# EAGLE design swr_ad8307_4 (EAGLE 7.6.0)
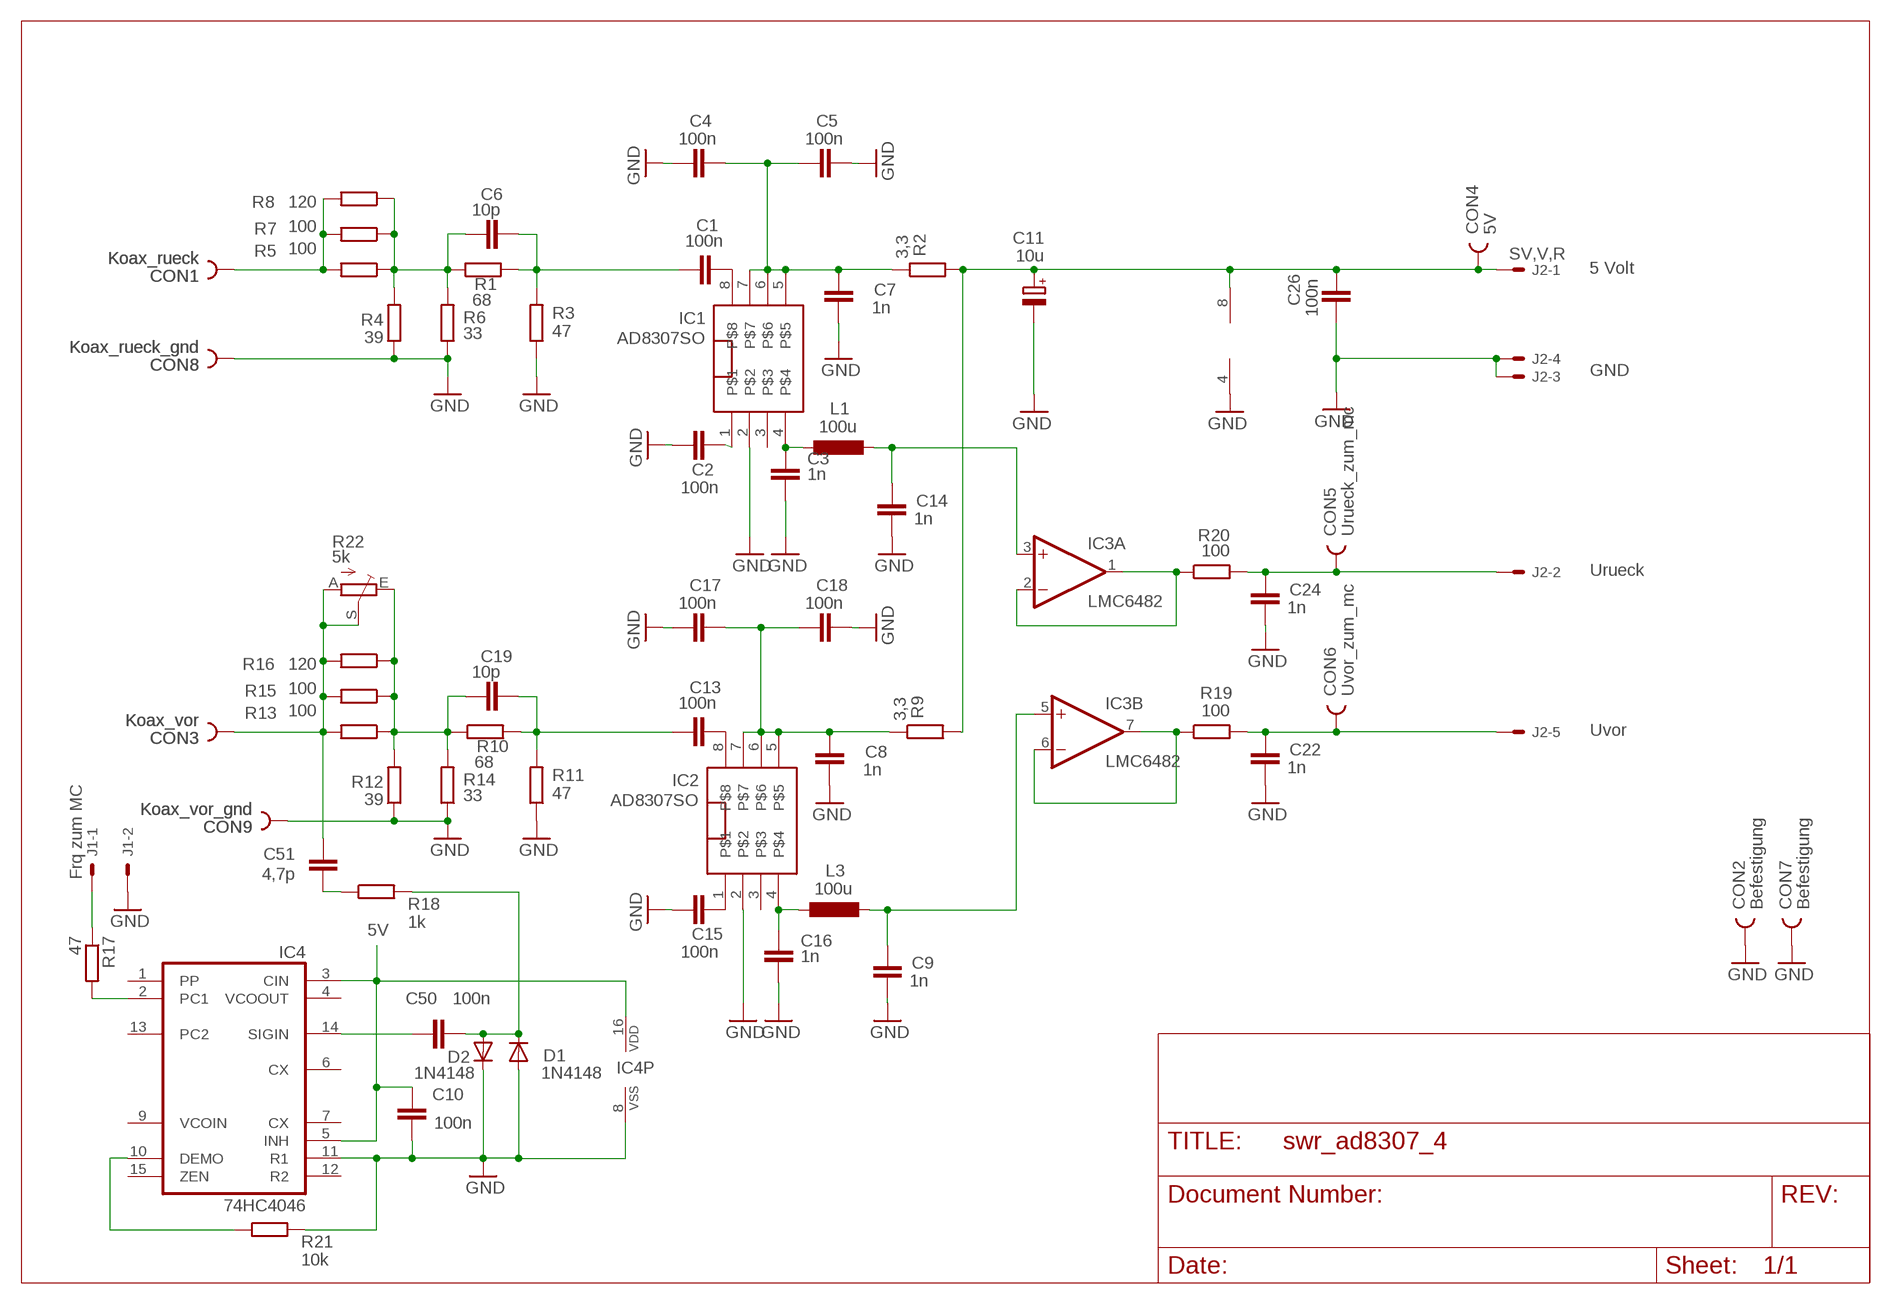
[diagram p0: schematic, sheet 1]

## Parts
C1  100n  C-EUC0805  [C0805]
C2  100n  C-EUC0805  [C0805]
C3  1n  C-EUC0805  [C0805]
C4  100n  C-EUC0805  [C0805]
C5  100n  C-EUC0805  [C0805]
C6  10p  C-EUC0805  [C0805]
C7  1n  C-EUC0805  [C0805]
C8  1n  C-EUC0805  [C0805]
C9  1n  C-EUC0805  [C0805]
C10  100n  C-EUC0805  [C0805]
C11  10u  CPOL-EUSMCB  [SMC_B]
C13  100n  C-EUC0805  [C0805]
C14  1n  C-EUC0805  [C0805]
C15  100n  C-EUC0805  [C0805]
C16  1n  C-EUC0805  [C0805]
C17  100n  C-EUC0805  [C0805]
C18  100n  C-EUC0805  [C0805]
C19  10p  C-EUC0805  [C0805]
C22  1n  C-EUC0805  [C0805]
C24  1n  C-EUC0805  [C0805]
C26  100n  C-EUC0805  [C0805]
C50  100n  C-EUC0805  [C0805]
C51  4,7p  C-EUC0805  [C0805]
CON1  Koax_rueck  PIN1_75OV  [PIN_1,75OV]
CON2  Befestigung  PIN2_53MM  [HOLE3]
CON3  Koax_vor  PIN1_75OV  [PIN_1,75OV]
CON4  5V  PIN1_75  [PIN1_75]
CON5  Urueck_zum_mc  PIN1_75  [PIN1_75]
CON6  Uvor_zum_mc  PIN1_75  [PIN1_75]
CON7  Befestigung  PIN2_53MM  [HOLE3]
CON8  Koax_rueck_gnd  PIN1_75OV  [PIN_1,75OV]
CON9  Koax_vor_gnd  PIN1_75OV  [PIN_1,75OV]
D1  1N4148  DIODE-SOD80C  [SOD80C]
D2  1N4148  DIODE-SOD80C  [SOD80C]
IC1  AD8307SO  [SO8]
IC2  AD8307SO  [SO8]
IC3  LMC6482  TL082D  [SO08]
IC4  74HC4046  4046D  [SO16]
J1  Frq zum MC  22-05-7028-02  [7395-02]
J2  SV,V,R  22-05-7058-05  [7395-05]
L1  100u  L-EUL3230M  [L3230M]
L3  100u  L-EUL3230M  [L3230M]
R1  68  R-EU_M0805  [M0805]
R2  3,3  R-EU_M0805  [M0805]
R3  47  R-EU_M0805  [M0805]
R4  39  R-EU_M0805  [M0805]
R5  100  R-EU_M1206  [M1206]
R6  33  R-EU_M0805  [M0805]
R7  100  R-EU_M1206  [M1206]
R8  120  R-EU_M1206  [M1206]
R9  3,3  R-EU_M0805  [M0805]
R10  68  R-EU_M0805  [M0805]
R11  47  R-EU_M0805  [M0805]
R12  39  R-EU_M0805  [M0805]
R13  100  R-EU_M1206  [M1206]
R14  33  R-EU_M0805  [M0805]
R15  100  R-EU_M1206  [M1206]
R16  120  R-EU_M1206  [M1206]
R17  47  R-EU_M0805  [M0805]
R18  1k  R-EU_M0805  [M0805]
R19  100  R-EU_M0805  [M0805]
R20  100  R-EU_M0805  [M0805]
R21  10k  R-EU_M0805  [M0805]
R22  5k  TRIM_EU-CA6H  [CA6H]

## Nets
5V: C10.2 C11.+ C26.1 CON4.1 IC3.8(P:V+) IC4.3(CIN) IC4.5(INH) IC4.16(VDD) J2.1 R2.2 R9.2
GND: C2.1 C3.1 C4.2 C5.1 C7.2 C8.2 C9.2 C10.1 C11.- C14.2 C15.1 C16.1 C17.2 C18.1 C22.2 C24.2 C26.2 CON2.1 CON7.1 CON8.1 CON9.1 D1.A D2.C IC1.2 IC2.2 IC3.4(P:V-) IC4.8(VSS) IC4.11(R1) J1.2 J2.3 J2.4 R3.1 R4.1 R6.1 R11.1 R12.1 R14.1 R21.2
N$1: C1.2 IC1.8
N$2: IC4.10(DEMO) R21.1
N$3: C2.2 IC1.1
N$4: C4.1 C5.2 C7.1 IC1.5 IC1.6 IC1.7 R2.1
N$5: CON1.1 R5.2 R7.2 R8.2
N$6: C16.2 IC2.4 L3.1
N$7: C1.1 C6.2 R1.2 R3.2
N$8: IC3.6(B:-IN) IC3.7(B:OUT) R19.1
N$9: C6.1 R1.1 R4.2 R5.1 R6.2 R7.1 R8.1
N$10: IC3.1(A:OUT) IC3.2(A:-IN) R20.1
N$11: C3.2 IC1.4 L1.1
N$12: IC4.2(PC1) R17.2
N$14: C14.1 IC3.3(A:+IN) L1.2
N$15: C9.1 IC3.5(B:+IN) L3.2
N$16: C13.2 IC2.8
N$17: C15.2 IC2.1
N$18: C8.1 C17.1 C18.2 IC2.5 IC2.6 IC2.7 R9.1
N$19: C51.2 CON3.1 R13.2 R15.2 R16.2 R22.A R22.S
N$20: C13.1 C19.2 R10.2 R11.2
N$22: C19.1 R10.1 R12.2 R13.1 R14.2 R15.1 R16.1 R22.E
N$28: C22.1 CON6.1 J2.5 R19.2
N$29: J1.1 R17.1
N$30: C24.1 CON5.1 J2.2 R20.2
N$77: C50.1 IC4.14(SIGIN)
N$78: C50.2 D1.C D2.A R18.2
N$79: C51.1 R18.1
Unconnected: IC1.3 IC2.3 IC4.1(PP) IC4.4(VCOOUT) IC4.6(CX) IC4.7(CX) IC4.9(VCOIN) IC4.12(R2) IC4.13(PC2) IC4.15(ZEN)

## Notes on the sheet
- 5 Volt
- GND
- Urueck
- Uvor

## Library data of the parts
C1-C10 C13-C19 C22 C24 C26 C50 C51 = rcl:C-EU: CAPACITOR, European symbol
C11 = rcl:CPOL-EU: POLARIZED CAPACITOR, European symbol
CON1 CON3-CON6 CON8 CON9 = lindenau:PIN1_75
CON2 CON7 = lindenau:PIN2_5
D1 D2 = diode:DIODE-: DIODE
IC1 IC2 = analog-devices1:AD8307
IC3 = linear:TL082: OP AMP
IC4 = 40xx:4046: Micropower PLL
J1 = con-molex:22-?-02: CONNECTOR; OC_FARNELL: 9731601; OC_NEWARK: unknown
J2 = con-molex:22-?-05: CONNECTOR wire to board 2.54 mm (.1 inch) pitch header; OC_FARNELL: unknown; OC_NEWARK: unknown
L1 L3 = rcl:L-EU: INDUCTOR, European symbol
R1-R21 = rcl:R-EU_: RESISTOR, European symbol
R22 = pot:TRIM_EU-: POTENTIOMETER

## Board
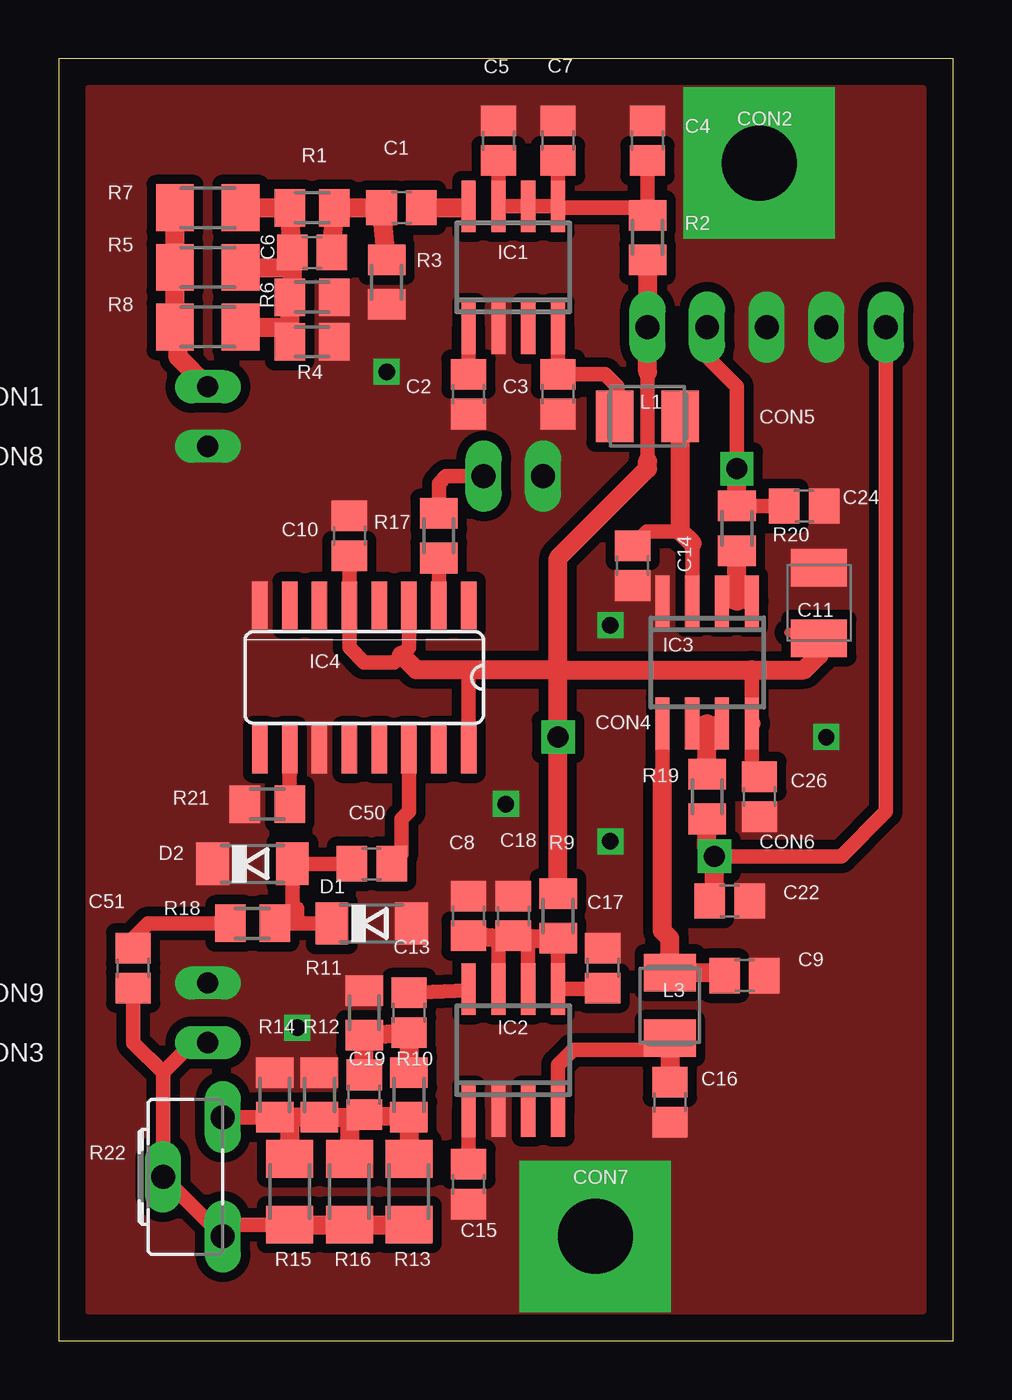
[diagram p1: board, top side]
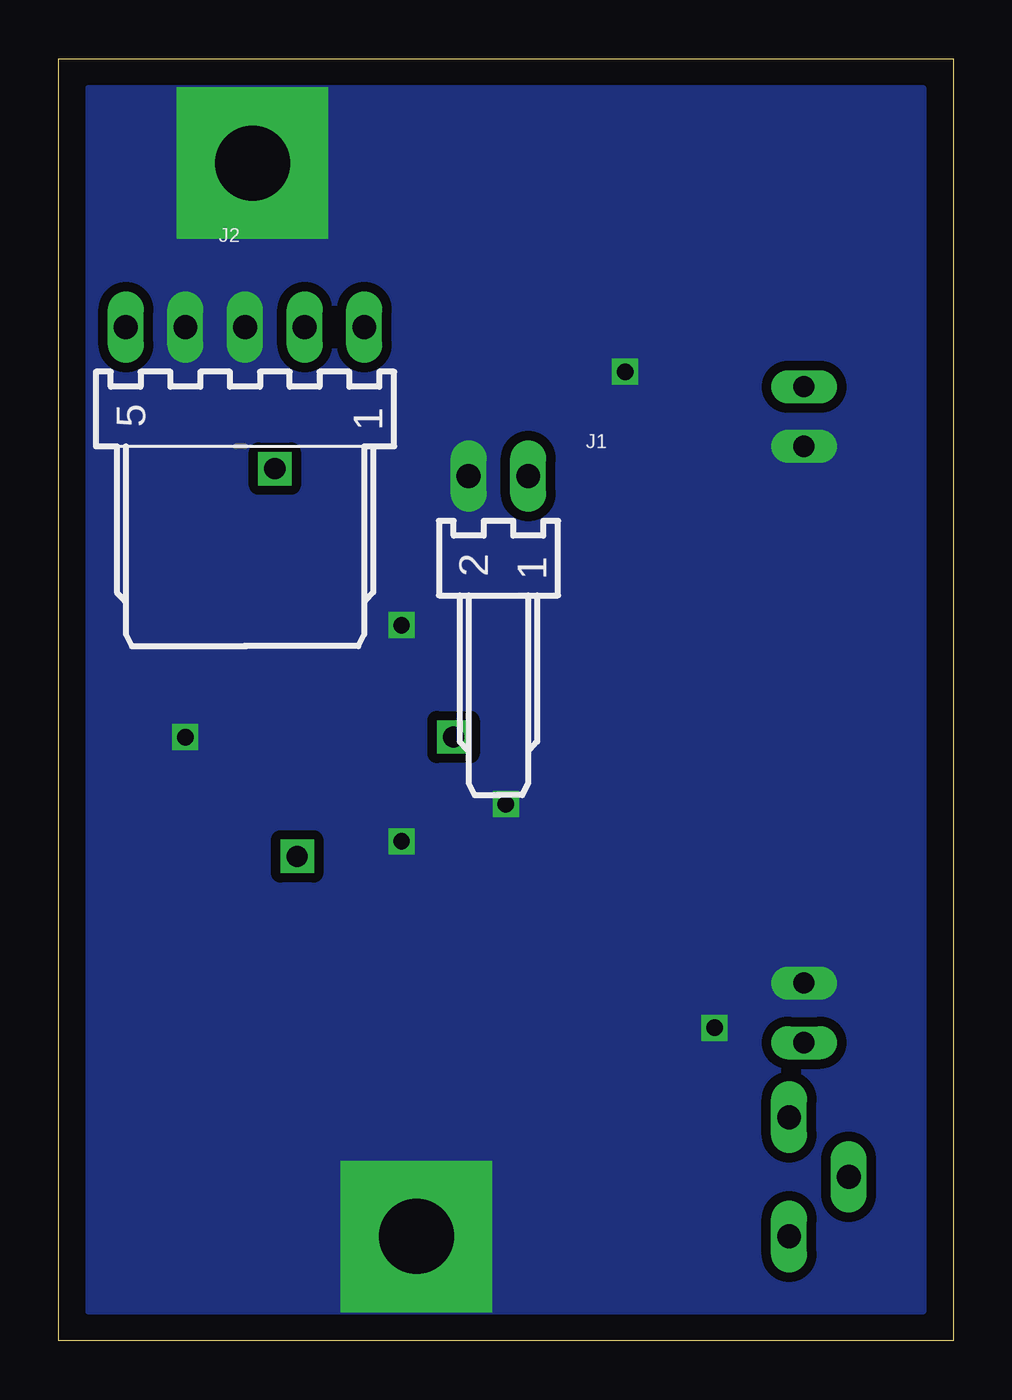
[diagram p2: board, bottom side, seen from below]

Size 38.1 x 54.61 mm. Coordinates in mm from the lower left corner, seen from the top.
Outline: 0,0 38.1,0 38.1,54.61 0,54.61 0,0
Copper layers (1*16): Top 0.035mm / dielectric 1.5mm / Bottom 0.035mm
Design rules "default": minimum track width 10mil, minimum drill 24mil, track to track 8mil, track to pad 8mil, pad to pad 8mil, via to via 8mil, smd to smd 8mil, copper to edge 40mil, drill to drill 8mil, minimum pad ring 10mil, minimum via ring 8mil, stop-mask expansion 4mil, vias tented up to drill 0mil, thermal gap 10mil

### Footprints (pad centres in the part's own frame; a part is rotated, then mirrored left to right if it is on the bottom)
C0805 = smd 1.3 x 1.5: 1 -0.85,0; 2 0.85,0
SMC_B = smd 1.6 x 2.4: + -1.5,0; - 1.5,0
PIN_1,75OV = drill 0.9 pad 1.397 long: 1 0,0
HOLE3 = drill 3.2 pad 6.452 square: 1 0,0
PIN1_75 = drill 0.9 pad 1.422 square: 1 0,0
SOD80C = smd 1.4 x 1.8: A 1.7,0; C -1.7,0
SO8 = smd 0.6 x 2.2: 1 -1.905,-2.6; 2 -0.635,-2.6; 3 0.635,-2.6; 4 1.905,-2.6; 5 1.905,2.6; 6 0.635,2.6; 7 -0.635,2.6; 8 -1.905,2.6
SO08 = smd 0.6 x 2.2: 1 -1.905,-2.6; 2 -0.635,-2.6; 3 0.635,-2.6; 4 1.905,-2.6; 5 1.905,2.6; 6 0.635,2.6; 7 -0.635,2.6; 8 -1.905,2.6
SO16 = smd 0.66 x 2.032: 1 -4.445,-3.073; 2 -3.175,-3.073; 3 -1.905,-3.073; 4 -0.635,-3.073; 5 0.635,-3.073; 6 1.905,-3.073; 7 3.175,-3.073; 8 4.445,-3.073; 9 4.445,3.073; 10 3.175,3.073; 11 1.905,3.073; 12 0.635,3.073; 13 -0.635,3.073; 14 -1.905,3.073; 15 -3.175,3.073; 16 -4.445,3.073
7395-02 = drill 1.016 long: 1 1.27,0; 2 -1.27,0
7395-05 = drill 1.016 long: 1 5.08,0; 2 2.54,0; 3 0,0; 4 -2.54,0; 5 -5.08,0
L3230M = smd 1.6 x 2.2: 1 -1.4,0; 2 1.4,0
M0805 = smd 1.3 x 1.6: 1 -0.95,0; 2 0.95,0
M1206 = smd 1.6 x 2: 1 -1.4,0; 2 1.4,0
CA6H = drill 1.016 long: A -2.54,0; E 2.54,0; S 0,2.54

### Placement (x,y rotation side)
C1  14.61,48.26 0 top
C2  17.46,40.32 90 top
C3  21.27,40.32 90 top
C4  25.08,51.12 90 top
C5  18.73,51.12 270 top
C6  10.79,46.36 0 top
C7  21.27,51.12 90 top
C8  17.46,18.1 90 top
C9  29.21,15.56 0 top
C10  12.38,34.29 270 top
C11  32.38,31.43 90 top
C13  14.92,13.97 90 top
C14  24.45,33.02 270 top
C15  17.46,6.67 90 top
C16  26.04,10.16 90 top
C17  23.18,15.88 90 top
C18  19.37,18.1 270 top
C19  13.02,10.48 90 top
C22  28.57,18.73 0 top
C24  31.75,35.56 0 top
C26  29.84,23.18 270 top
C50  13.33,20.32 180 top
C51  3.17,15.88 270 top
CON1  6.35,40.64 180 top
CON2  29.84,50.17 0 top
CON3  6.35,12.7 180 top
CON4  21.27,25.72 90 top
CON5  28.89,37.15 180 top
CON6  27.94,20.64 180 top
CON7  22.86,4.45 0 top
CON8  6.35,38.1 180 top
CON9  6.35,15.24 180 top
D1  13.33,17.78 0 top
D2  8.26,20.32 0 top
IC1  19.37,45.72 0 top
IC2  19.37,12.38 0 top
IC3  27.62,28.89 180 top
IC4  13.02,28.26 180 top
J1  19.37,36.83 0 bottom
J2  30.16,43.18 0 bottom
L1  25.08,39.37 0 top
L3  26.04,14.29 90 top
R1  10.79,48.26 0 top
R2  25.08,46.99 270 top
R3  13.97,45.09 90 top
R4  10.79,42.55 180 top
R5  6.35,45.72 180 top
R6  10.79,44.45 180 top
R7  6.35,48.26 180 top
R8  6.35,43.18 180 top
R9  21.27,18.1 90 top
R10  14.92,10.48 90 top
R11  13.02,13.97 270 top
R12  11.11,10.48 270 top
R13  14.92,6.35 270 top
R14  9.21,10.48 270 top
R15  9.84,6.35 270 top
R16  12.38,6.35 270 top
R17  16.19,34.29 270 top
R18  8.26,17.78 0 top
R19  27.62,23.18 270 top
R20  28.89,34.61 90 top
R21  8.89,22.86 180 top
R22  6.98,6.98 90 top

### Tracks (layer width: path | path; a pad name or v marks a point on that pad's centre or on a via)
5V
  Top 0.406: C11.+ 31.11,30.16
  Top 0.61: 25.08,37.47 25.08,41.28 | IC4.3 14.92,29.53 14.61,29.21 14.29,28.89 13.02,28.89 12.38,29.53 IC4.5 C10.2 | 29.53,28.57 29.53,26.35 29.59,26.29 IC3.8 29.53,24.34 C26.1 | 17.46,28.57 IC4.16
  Top 0.813: R9.2 CON4.1 21.27,28.57 | 21.27,28.57 21.27,33.34 25.08,37.15 25.08,37.47 | 21.27,28.57 17.46,28.57 15.24,28.57 14.61,29.21 | 25.08,41.28 J2.1 R2.2 | 21.27,28.57 29.53,28.57 31.75,28.57 32.38,29.21 C11.+
GND  (via drill 0.7)
  other vias: 23.5,30.48 13.97,41.28 10.16,13.33 23.5,21.27 19.05,22.86 32.7,25.72
  pour Top (isolate 0.406, no thermals): 1.27,1.27 36.83,1.27 36.83,53.34 1.27,53.34
  pour Bottom (isolate 0.406, no thermals): 1.27,1.27 1.27,53.34 36.83,53.34 36.83,1.27
N$1
  Top 0.61: 17.14,48.26 IC1.8
  Top 0.813: C1.2 17.14,48.26
N$2
  Top 0.61: R21.1 9.84,24.55 IC4.10
N$3
  Top 0.61: C2.2 IC1.1
N$4
  Top 0.61: C5.2 IC1.7 IC1.6 IC1.5 | IC1.5 C7.1 | IC1.5 21.33,48.26 24.45,48.26 24.77,47.94 R2.1 C4.1
N$5
  Top 0.813: CON1.1 5.08,41.91 5.08,43.05 R8.2 R5.2 R7.2
N$6
  Top 0.61: IC2.4 21.27,11.75 21.91,12.38 25.53,12.38 L3.1
  Top 0.813: L3.1 C16.2
N$7
  Top 0.813: C6.2 R1.2 C1.1 R3.2
N$8
  Top 0.61: IC3.6 27.62,26.29 IC3.7
  Top 0.813: R19.1 27.62,26.29
N$9
  Top 0.813: R7.1 R1.1 C6.1 9.95,45.72 | 9.95,45.72 9.95,44.55 R6.2 9.84,43.18 | 9.84,43.18 R4.2 | R8.1 9.84,43.18 | R5.1 9.95,45.72
N$10
  Top 0.61: IC3.2 28.89,31.49 IC3.1
  Top 0.813: 28.89,31.49 R20.1
N$11
  Top 0.61: IC1.4 C3.2 23.28,41.17 23.81,40.64 23.81,39.5 L1.1
N$12
  Top 0.61: IC4.2 R17.2
N$14
  Top 0.61: IC3.3 26.99,33.97 | 26.48,34.48 25.05,34.48 C14.1
  Top 0.813: L1.2 26.48,34.48 26.99,33.97
N$15
  Top 0.61: 25.72,24.13 IC3.5
  Top 0.813: 25.72,24.13 25.72,17.46 26.04,17.14 L3.2 28.13,15.69 C9.1
N$16
  Top 0.61: C13.2 17.4,14.92 IC2.8
N$17
  Top 0.61: C15.2 IC2.1
N$18
  Top 0.61: IC2.7 18.73,17.15 | 20,17.15 IC2.6 | R9.1 IC2.5 23.12,14.98 C17.1
  Top 0.813: C8.1 18.73,17.15 C18.2 20,17.15 R9.1
N$19
  Top 0.61: R15.2 7.49,4.95 R22.A R22.S 4.45,11.43 | C51.2 3.17,12.7 4.45,11.43 | CON3.1 5.71,12.7 4.45,11.43
  Top 0.813: R15.2 R16.2 R13.2
N$20
  Top 0.813: C19.2 R11.2 C13.1 R10.2
N$22
  Top 0.61: R22.E R14.2
  Top 0.813: R13.1 R10.1 C19.1 12.38,9.53 | 12.38,9.53 R12.2 9.84,9.53 | 9.84,9.53 R14.2 | 9.84,9.53 R15.1 | 12.38,9.53 R16.1
N$28
  Top 0.61: J2.5 35.24,22.54 33.34,20.64 CON6.1
  Top 0.813: R19.2 27.62,20.95 CON6.1 27.94,18.95 C22.1
N$29
  Top 0.61: J1.1 16.51,36.83 16.19,36.51 R17.1
N$30
  Top 0.61: R20.2 30.58,35.56 C24.1 | J2.2 27.62,41.91 28.89,40.64 CON5.1
  Top 0.813: R20.2 CON5.1
N$77
  Top 0.61: IC4.14 14.92,22.54 14.61,22.22 14.61,20.74 C50.1
N$78
  Top 0.61: C50.2 D2.A 9.96,18.62 10.16,18.41 10.16,17.78 | R18.2 10.16,17.78 | 10.16,17.78 D1.C
N$79
  Top 0.61: R18.1 3.81,17.78 3.17,17.14 C51.1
